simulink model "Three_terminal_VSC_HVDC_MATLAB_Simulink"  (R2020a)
settings: Solver=ode4  StartTime=0.0  StopTime=Tstop  MaxStep=1e-4  RelTol=1e-3
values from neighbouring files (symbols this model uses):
  kw = 5    [Parameterisation_Three_terminal_VSC_HVDC_MATLAB_Simulink.m]
undefined symbols (not defined in the file or in its folder): bridge, phase, pulses, Sim, Three, VSC1, VSC123, VSC2, VSC3
libraries: powerlib x70, powerlib_meascontrol x9, simulink x3
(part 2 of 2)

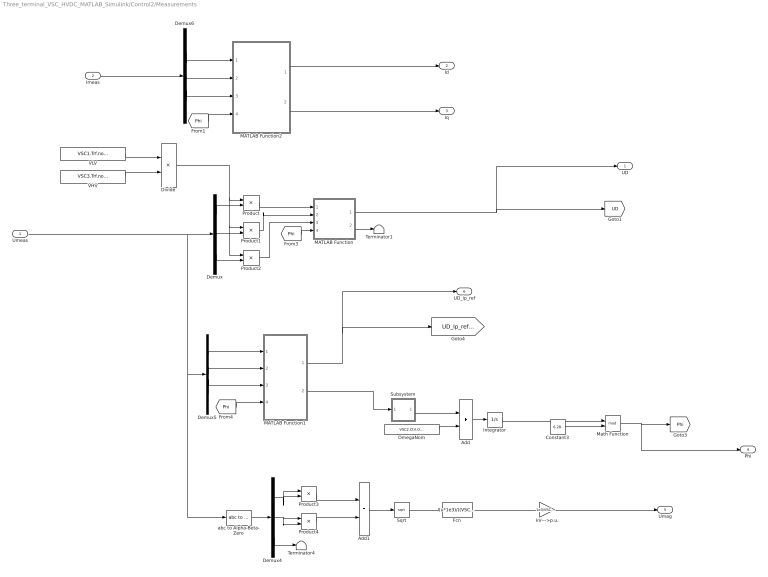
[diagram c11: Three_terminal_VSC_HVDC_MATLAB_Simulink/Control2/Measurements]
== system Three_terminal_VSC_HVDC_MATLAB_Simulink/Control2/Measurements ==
  Umeas : Inport
  Imeas : Inport  Port=2
  Add : Sum
  Add1 : Sum
  Constant3 : Constant  Value=6.28
  Demux{,4..6} (4 alike) : Demux  Outputs=3
  Divide : Product  Inputs=*/
  Fcn : Fcn  Expr=(u*1e3)/((VSC3.Trf.nominal.HV *sqrt(2))/(sqrt(3)*VSC3.Trf.nominal.HV ))/1000
  Integrator : Integrator
  MATLAB Function : MATLAB Function  TreatAsAtomicUnit=on
  MATLAB Function1 : MATLAB Function  TreatAsAtomicUnit=on
  MATLAB Function2 : MATLAB Function  TreatAsAtomicUnit=on
  Math Function : Math  Operator=mod
  OmegaNom : Constant  Value=VSC2.Ctrl.Omeganom
  Product{,1..4} (5 alike) : Product
  Sqrt : Sqrt
  Subsystem : Subsystem
  Terminator1 : Terminator
  Terminator4 : Terminator
  VHV : Constant  Value=VSC3.Trf.nominal.HV
  VLV : Constant  Value=VSC1.Trf.nominal.LV
  abc to Alpha-Beta-Zero : powerlib_meascontrol/Transformations/abc to Alpha-Beta-Zero
  kV--->p.u. : Gain  Gain=1e3/VSC3.Trf.nominal.HV
  UD : Outport
  Id : Outport  Port=2
  Iq : Outport  Port=3
  Phi : Outport  Port=4
  Umag : Outport  Port=5
  UD_ip_ref : Outport  Port=6
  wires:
  MATLAB Function1/2(xQ) -> Subsystem/1(Input)
  MATLAB Function2/2(xQ) -> Iq/1
  Demux/2 -> Product1/2
  Subsystem/1(Output) -> Add/1
  Math Function/1 -> Phi/1, [Phi]
  Product2/1 -> MATLAB Function/3(xC)
  Divide/1 -> Product/1, Product1/1, Product2/1
  Product/1 -> MATLAB Function/1(xA)
  VLV/1 -> Divide/1
  OmegaNom/1 -> Add/2
  Product1/1 -> MATLAB Function/2(xB)
  Add/1 -> Integrator/1
  VHV/1 -> Divide/2
  Demux/1 -> Product/2
  Demux/3 -> Product2/2
  MATLAB Function2/1(xD) -> Id/1
  abc to Alpha-Beta-Zero/1 -> Demux4/1
  Demux4/1 -> Product3/2, Product3/1
  Demux4/2 -> Product4/2, Product4/1
  Demux4/3 -> Terminator4/1
  Product3/1 -> Add1/1
  Product4/1 -> Add1/2
  Add1/1 -> Sqrt/1
  Sqrt/1 -> Fcn/1
  Fcn/1 -> kV--->p.u./1
  kV--->p.u./1 -> Umag/1
  Umeas/1 -> Demux/1, abc to Alpha-Beta-Zero/1, Demux5/1
  MATLAB Function1/1(xD) -> [UD_Ip_ref_cacl], UD_ip_ref/1
  Constant3/1 -> Math Function/2
  Integrator/1 -> Math Function/1
  [Phi] -> MATLAB Function/4(theta)
  MATLAB Function/1(xD) -> UD/1, [UD]
  [Phi] -> MATLAB Function1/4(theta)
  Demux5/1 -> MATLAB Function1/1(xA)
  Demux5/2 -> MATLAB Function1/2(xB)
  Demux5/3 -> MATLAB Function1/3(xC)
  Imeas/1 -> Demux6/1
  MATLAB Function/2(xQ) -> Terminator1/1
  Demux6/1 -> MATLAB Function2/1(xA)
  Demux6/2 -> MATLAB Function2/2(xB)
  Demux6/3 -> MATLAB Function2/3(xC)
  [Phi] -> MATLAB Function2/4(theta)

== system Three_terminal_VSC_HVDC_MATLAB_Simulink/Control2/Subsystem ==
  Input : Inport
  Add : Sum
  Add1 : Sum  Inputs=-+
  Add2 : Sum
  Gain : Gain  Gain=VSC1.Ctrl.AC.Kp
  Gain1 : Gain  Gain=kw
  Gain2 : Gain  Gain=VSC2.Ctrl.AC.Ti
  Integrator : Integrator
  Saturation : Saturate  UpperLimit=VSC1.Ctrl.Iqmax  LowerLimit=VSC1.Ctrl.Iqmin
  Output : Outport
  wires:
  Gain/1 -> Add/1
  Input/1 -> Add2/1, Gain/1
  Add/1 -> Add1/1, Saturation/1
  Saturation/1 -> Add1/2, Output/1
  Add1/1 -> Gain1/1
  Gain1/1 -> Add2/2
  Add2/1 -> Gain2/1
  Gain2/1 -> Integrator/1
  Integrator/1 -> Add/2

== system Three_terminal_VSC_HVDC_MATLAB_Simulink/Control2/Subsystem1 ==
  Input : Inport
  Add : Sum
  Add1 : Sum  Inputs=-+
  Add2 : Sum
  Gain : Gain  Gain=VSC1.Ctrl.DC.Kp
  Gain1 : Gain  Gain=kw
  Gain2 : Gain  Gain=VSC2.Ctrl.DC.Ti
  Integrator : Integrator
  Saturation : Saturate  UpperLimit=VSC1.Ctrl.Idmax  LowerLimit=VSC1.Ctrl.Idmin
  Output : Outport
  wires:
  Gain/1 -> Add/1
  Input/1 -> Add2/1, Gain/1
  Add/1 -> Add1/1, Saturation/1
  Saturation/1 -> Add1/2, Output/1
  Add1/1 -> Gain1/1
  Gain1/1 -> Add2/2
  Add2/1 -> Gain2/1
  Gain2/1 -> Integrator/1
  Integrator/1 -> Add/2

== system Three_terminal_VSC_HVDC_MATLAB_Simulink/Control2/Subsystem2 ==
  Input : Inport
  Add : Sum
  Add1 : Sum  Inputs=-+
  Add2 : Sum
  Gain : Gain  Gain=VSC1.Ctrl.Current.Kp
  Gain1 : Gain  Gain=kw
  Gain2 : Gain  Gain=VSC1.Ctrl.Current.Ti
  Integrator : Integrator
  Saturation : Saturate  UpperLimit=VSC1.Ctrl.Umax  LowerLimit=VSC1.Ctrl.Umin
  Output : Outport
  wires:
  Gain/1 -> Add/1
  Input/1 -> Add2/1, Gain/1
  Add/1 -> Add1/1, Saturation/1
  Saturation/1 -> Add1/2, Output/1
  Add1/1 -> Gain1/1
  Gain1/1 -> Add2/2
  Add2/1 -> Gain2/1
  Gain2/1 -> Integrator/1
  Integrator/1 -> Add/2

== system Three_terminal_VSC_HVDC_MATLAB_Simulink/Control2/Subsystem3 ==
  Input : Inport
  Add : Sum
  Add1 : Sum  Inputs=-+
  Add2 : Sum
  Gain : Gain  Gain=VSC1.Ctrl.Current.Kp
  Gain1 : Gain  Gain=kw
  Gain2 : Gain  Gain=VSC1.Ctrl.Current.Ti
  Integrator : Integrator
  Saturation : Saturate  UpperLimit=VSC1.Ctrl.Umax  LowerLimit=VSC1.Ctrl.Umin
  Output : Outport
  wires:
  Gain/1 -> Add/1
  Input/1 -> Add2/1, Gain/1
  Add/1 -> Add1/1, Saturation/1
  Saturation/1 -> Add1/2, Output/1
  Add1/1 -> Gain1/1
  Gain1/1 -> Add2/2
  Add2/1 -> Gain2/1
  Gain2/1 -> Integrator/1
  Integrator/1 -> Add/2

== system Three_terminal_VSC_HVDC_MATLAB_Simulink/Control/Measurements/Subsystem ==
  Input : Inport
  Add : Sum
  Add1 : Sum  Inputs=-+
  Add2 : Sum
  Gain : Gain  Gain=VSC1.Ctrl.PLL.PI.Kp
  Gain1 : Gain  Gain=kw
  Gain2 : Gain  Gain=VSC1.Ctrl.PLL.PI.Ti
  Integrator : Integrator
  Saturation : Saturate  UpperLimit=VSC1.Ctrl.Deltaomegamax  LowerLimit=VSC1.Ctrl.Deltaomegamin
  Output : Outport
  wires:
  Gain/1 -> Add/1
  Input/1 -> Add2/1, Gain/1
  Add/1 -> Add1/1, Saturation/1
  Saturation/1 -> Add1/2, Output/1
  Add1/1 -> Gain1/1
  Gain1/1 -> Add2/2
  Add2/1 -> Gain2/1
  Gain2/1 -> Integrator/1
  Integrator/1 -> Add/2

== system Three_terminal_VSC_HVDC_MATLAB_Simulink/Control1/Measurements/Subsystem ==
  Input : Inport
  Add : Sum
  Add1 : Sum  Inputs=-+
  Add2 : Sum
  Gain : Gain  Gain=VSC1.Ctrl.PLL.PI.Kp
  Gain1 : Gain  Gain=kw
  Gain2 : Gain  Gain=VSC1.Ctrl.PLL.PI.Ti
  Integrator : Integrator
  Saturation : Saturate  UpperLimit=VSC1.Ctrl.Deltaomegamax  LowerLimit=VSC1.Ctrl.Deltaomegamin
  Output : Outport
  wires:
  Gain/1 -> Add/1
  Input/1 -> Add2/1, Gain/1
  Add/1 -> Add1/1, Saturation/1
  Saturation/1 -> Add1/2, Output/1
  Add1/1 -> Gain1/1
  Gain1/1 -> Add2/2
  Add2/1 -> Gain2/1
  Gain2/1 -> Integrator/1
  Integrator/1 -> Add/2

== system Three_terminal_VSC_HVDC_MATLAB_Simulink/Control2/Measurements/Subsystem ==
  Input : Inport
  Add : Sum
  Add1 : Sum  Inputs=-+
  Add2 : Sum
  Gain : Gain  Gain=VSC1.Ctrl.PLL.PI.Kp
  Gain1 : Gain  Gain=kw
  Gain2 : Gain  Gain=VSC1.Ctrl.PLL.PI.Ti
  Integrator : Integrator
  Saturation : Saturate  UpperLimit=VSC1.Ctrl.Deltaomegamax  LowerLimit=VSC1.Ctrl.Deltaomegamin
  Output : Outport
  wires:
  Gain/1 -> Add/1
  Input/1 -> Add2/1, Gain/1
  Add/1 -> Add1/1, Saturation/1
  Saturation/1 -> Add1/2, Output/1
  Add1/1 -> Gain1/1
  Gain1/1 -> Add2/2
  Add2/1 -> Gain2/1
  Gain2/1 -> Integrator/1
  Integrator/1 -> Add/2

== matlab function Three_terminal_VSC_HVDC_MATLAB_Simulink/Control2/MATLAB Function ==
function [xA,xB,xC] = fcn(Pmd,Pmq,theta)

xA = cos(theta)*Pmd           - sin(theta)*Pmq            +  1*0;

xB = cos(theta-2*pi()/3)*Pmd  - sin(theta-2*pi()/3)*Pmq   +  1*0;

xC = cos(theta+2*pi()/3)*Pmd  - sin(theta+2*pi()/3)*Pmq   +  1*0;

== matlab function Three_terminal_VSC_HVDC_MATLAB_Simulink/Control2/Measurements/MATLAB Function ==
function [xD,xQ] = fcn(xA,xB,xC,theta)

xD = (2/3*(cos(theta)*xA + cos(theta-2*pi()/3)*xB + cos(theta+2*pi()/3)*xC));

xQ = (2/3*(-sin(theta)*xA  - sin(theta-2*pi()/3)*xB   -  sin(theta+2*pi()/3)*xC));

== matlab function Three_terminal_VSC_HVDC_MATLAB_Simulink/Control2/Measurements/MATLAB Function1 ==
function [xD,xQ] = fcn(xA,xB,xC,theta)

xD = (2/3*(cos(theta)*xA + cos(theta-2*pi()/3)*xB + cos(theta+2*pi()/3)*xC));

xQ = (2/3*(-sin(theta)*xA  - sin(theta-2*pi()/3)*xB   -  sin(theta+2*pi()/3)*xC));

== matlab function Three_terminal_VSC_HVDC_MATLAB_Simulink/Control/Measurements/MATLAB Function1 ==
function [xD,xQ] = fcn(xA,xB,xC,theta)

xD = (2/3*(cos(theta)*xA + cos(theta-2*pi()/3)*xB + cos(theta+2*pi()/3)*xC));

xQ = (2/3*(-sin(theta)*xA  - sin(theta-2*pi()/3)*xB   -  sin(theta+2*pi()/3)*xC));

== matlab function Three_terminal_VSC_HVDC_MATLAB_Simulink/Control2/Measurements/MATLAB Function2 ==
function [xD,xQ] = fcn(xA,xB,xC,theta)

xD = (2/3*(cos(theta)*xA + cos(theta-2*pi()/3)*xB + cos(theta+2*pi()/3)*xC));

xQ = (2/3*(-sin(theta)*xA  - sin(theta-2*pi()/3)*xB   -  sin(theta+2*pi()/3)*xC));

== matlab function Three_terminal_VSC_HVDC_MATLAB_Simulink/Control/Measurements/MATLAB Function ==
function [xD,xQ] = fcn(xA,xB,xC,theta)

xD = (2/3*(cos(theta)*xA + cos(theta-2*pi()/3)*xB + cos(theta+2*pi()/3)*xC));

xQ = (2/3*(-sin(theta)*xA  - sin(theta-2*pi()/3)*xB   -  sin(theta+2*pi()/3)*xC));

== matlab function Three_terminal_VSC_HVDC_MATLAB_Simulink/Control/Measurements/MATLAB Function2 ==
function [xD,xQ] = fcn(xA,xB,xC,theta)

xD = (2/3*(cos(theta)*xA + cos(theta-2*pi()/3)*xB + cos(theta+2*pi()/3)*xC));

xQ = (2/3*(-sin(theta)*xA  - sin(theta-2*pi()/3)*xB   -  sin(theta+2*pi()/3)*xC));

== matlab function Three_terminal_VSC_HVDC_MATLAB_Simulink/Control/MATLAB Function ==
function [xA,xB,xC] = fcn(Pmd,Pmq,theta)

xA = cos(theta)*Pmd           - sin(theta)*Pmq            +  1*0;

xB = cos(theta-2*pi()/3)*Pmd  - sin(theta-2*pi()/3)*Pmq   +  1*0;

xC = cos(theta+2*pi()/3)*Pmd  - sin(theta+2*pi()/3)*Pmq   +  1*0;

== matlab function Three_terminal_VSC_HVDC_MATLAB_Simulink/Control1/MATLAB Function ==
function [xA,xB,xC] = fcn(Pmd,Pmq,theta)

xA = cos(theta)*Pmd           - sin(theta)*Pmq            +  1*0;

xB = cos(theta-2*pi()/3)*Pmd  - sin(theta-2*pi()/3)*Pmq   +  1*0;

xC = cos(theta+2*pi()/3)*Pmd  - sin(theta+2*pi()/3)*Pmq   +  1*0;

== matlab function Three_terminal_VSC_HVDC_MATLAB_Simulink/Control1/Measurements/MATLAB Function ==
function [xD,xQ] = fcn(xA,xB,xC,theta)

xD = (2/3*(cos(theta)*xA + cos(theta-2*pi()/3)*xB + cos(theta+2*pi()/3)*xC));

xQ = (2/3*(-sin(theta)*xA  - sin(theta-2*pi()/3)*xB   -  sin(theta+2*pi()/3)*xC));

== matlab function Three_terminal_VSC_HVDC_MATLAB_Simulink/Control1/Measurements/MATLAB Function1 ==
function [xD,xQ] = fcn(xA,xB,xC,theta)

xD = (2/3*(cos(theta)*xA + cos(theta-2*pi()/3)*xB + cos(theta+2*pi()/3)*xC));

xQ = (2/3*(-sin(theta)*xA  - sin(theta-2*pi()/3)*xB   -  sin(theta+2*pi()/3)*xC));

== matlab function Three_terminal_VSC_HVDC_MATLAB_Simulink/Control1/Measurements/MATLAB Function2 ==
function [xD,xQ] = fcn(xA,xB,xC,theta)

xD = (2/3*(cos(theta)*xA + cos(theta-2*pi()/3)*xB + cos(theta+2*pi()/3)*xC));

xQ = (2/3*(-sin(theta)*xA  - sin(theta-2*pi()/3)*xB   -  sin(theta+2*pi()/3)*xC));
